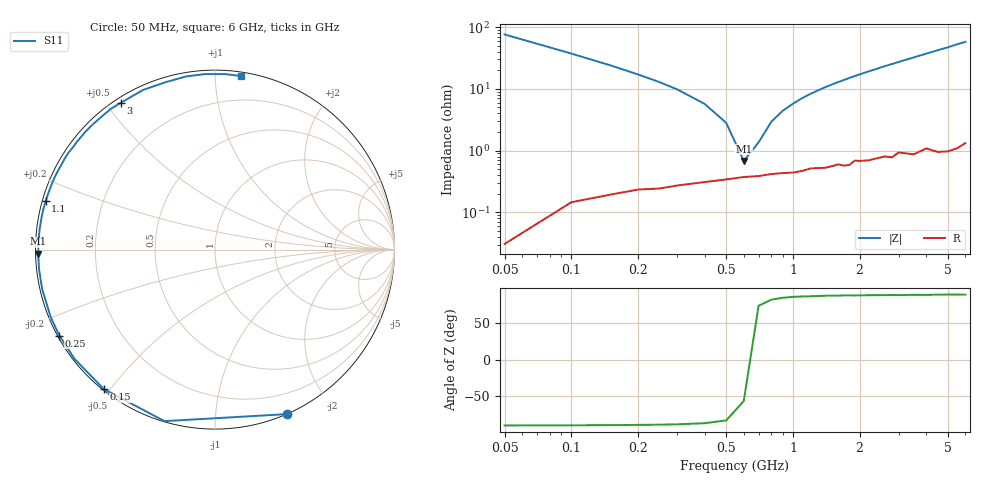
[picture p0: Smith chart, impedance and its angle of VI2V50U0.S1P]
! Infineon Technologies  Discrete & RF Semiconductors
! BB 804
! Si Tuning Diode in SOT23
! VR = 2.5 V
! S-Parameters:  July  1999
# GHz  S  MA  R  50
!  f  S11
! GHz  MAG  ANG
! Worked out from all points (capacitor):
!   34 points, 50 MHz to 6 GHz, reference 50 ohm
!   read as one part to ground: C = 41.5 pF near 50 MHz
!   lowest |Z| = 679 mohm at 600 MHz (marker M1)
!   series resonance near 630.2 MHz, so ESL is about 1.5 nH
!   S11 on the Smith chart (normalised r, x): 50 MHz: 0.00, -1.53; 150 MHz: 0.00, -0.48; 250 MHz: 0.00, -0.26; 1.1 GHz: 0.01, +0.14; 3 GHz: 0.02, +0.55; 6 GHz: 0.03, +1.16
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0.05  0.9996 -66.5
0.1  0.9963 -106.4
0.15  0.9937 -128.5
0.2  0.9917 -142.1
0.25  0.9909 -151.1
0.3  0.9896 -157.7
0.4  0.9879 -167.0
0.5  0.9865 -173.6
0.6  0.9852 -178.7
0.7  0.9846 177.0
0.8  0.9835 173.3
0.9  0.983 169.9
1.1  0.9818 163.9
1.4  0.98 155.9
1.6  0.9778 151.1
1.8  0.9787 146.4
2  0.9759 142.1
2.2  0.976 137.8
2.4  0.9748 134.0
2.6  0.9739 129.8
2.8  0.9755 126.3
3  0.9716 122.6
3.5  0.9757 114.3
4  0.9725 106.5
4.5  0.9781 99.5
5  0.9796 93.3
5.5  0.9796 86.8
6  0.9776 81.6
